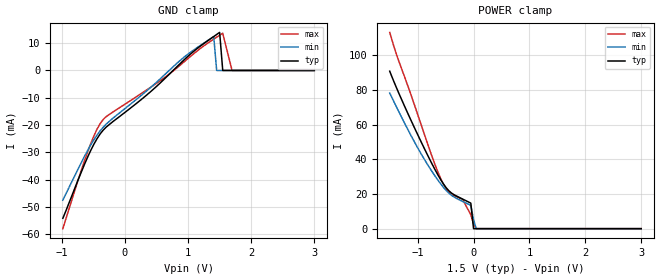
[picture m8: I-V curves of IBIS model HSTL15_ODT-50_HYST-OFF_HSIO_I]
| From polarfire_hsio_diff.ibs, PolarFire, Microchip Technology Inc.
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|   Model HSTL15_ODT-50_HYST-OFF_HSIO_I
[Model]   HSTL15_ODT-50_HYST-OFF_HSIO_I
Model_type   Input
Vinl =   0.65
Vinh =   0.85
|   typ   min   max
C_comp_pullup   1.335e-12   1.335e-12   1.380e-12
C_comp_pulldown  1.335e-12   1.335e-12   1.380e-12
[Temperature Range]  25C   100C   -40C
[Voltage Range]  1.5   1.425   1.575
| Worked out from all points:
|   POWER clamp passes 1 mA (typ) near -0.00 V on its own axis
[GND Clamp]
| Voltage   I(typ)   I(min)   I(max)
-984.4mV  -54.1mA    -47.47mA   -57.9mA
-590.6mV  -31.66mA   -29.23mA   -29.75mA
-443mV    -24.97mA   -23.63mA   -21.5mA
-344.5mV  -21.82mA   -20.76mA   -17.92mA
421.9mV   -7.443mA   -5.917mA   -5.928mA
937.5mV   3.9mA      4.886mA    3.178mA
1.406V    12.43mA    12.4mA     11.48mA
1.453V    13.18mA    0A         12.19mA
1.5V      13.94mA    0A         12.89mA
1.549V    0A         0A         13.63mA
1.697V    0A         0A         0A
3V        0A         0A         0A
[POWER Clamp]
| Voltage   I(typ)   I(min)   I(max)
-1.5V     90.81mA    78.21mA    113.2mA
-1.378V   81.18mA    70.13mA    100.4mA
-1.034V   56.55mA    48.6mA     69.11mA
-738.3mV  37.05mA    32.72mA    41.23mA
-590.6mV  28.4mA     25.94mA    29.11mA
-492.2mV  23.7mA     22.11mA    23.21mA
-443mV    21.89mA    20.52mA    21.28mA
-196.9mV  17.08mA    15.72mA    16.94mA
-49.22mV  14.73mA    13.45mA    8.041mA
0V        0A         5.249mA    2.764mA
46.88mV   0A         0A         0A
3V        0A         0A         0A
